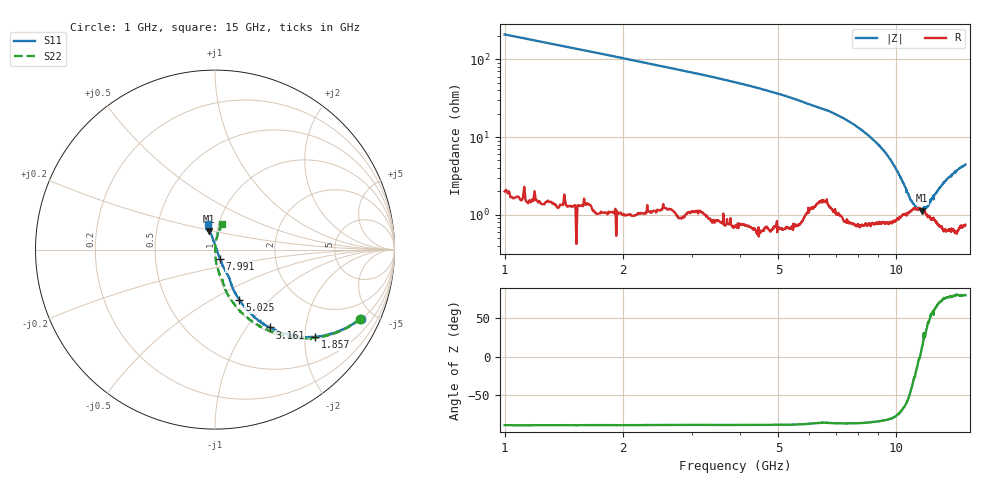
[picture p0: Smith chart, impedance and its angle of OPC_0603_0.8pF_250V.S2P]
! FILE NAME
! DATE 08/21/2012  14:12
! CORRECTED  DATA
# GHz  S  MA  R  50.00
!  FREQ  S11M  S11A  S21M  S21A  S12M  S12A  S22M  S22A
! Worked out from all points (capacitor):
!   1601 points, 1 GHz to 15 GHz, reference 50 ohm
!   read as one part in series: C = 748 fF near 1.07 GHz
!   lowest |Z| = 1.13 ohm at 11.61 GHz (marker M1)
!   series resonance near 11.49 GHz, so ESL is about 260 pH
!   S11 on the Smith chart (normalised r, x): 1 GHz: 1.06, -4.20; 1.857 GHz: 1.05, -2.26; 3.161 GHz: 1.07, -1.29; 5.025 GHz: 1.09, -0.68; 7.991 GHz: 1.05, -0.11; 15 GHz: 0.89, +0.26
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1  0.8978 -25.3  0.429 64.1  0.4288 64.0  0.8982 -25.5
1.8575  0.7409 -41.0  0.6622 48.2  0.662 48.2  0.7406 -41.6
3.16125  0.5303 -54.8  0.8365 33.2  0.8361 33.1  0.5295 -57.2
3.33625  0.5081 -56.2  0.8521 31.8  0.8514 31.8  0.5065 -58.8
5.025  0.3114 -64.1  0.9418 21.5  0.9416 21.5  0.3109 -71.2
5.6725  0.2457 -65.4  0.9599 18.6  0.9598 18.6  0.2444 -75.0
7.0375  0.1348 -64.1  0.9797 14.5  0.9792 14.4  0.132 -80.1
7.99125  0.05972 -61.9  0.9894 11.8  0.988 11.9  0.05897 -85.3
8  0.05941 -61.3  0.9893 11.8  0.988 11.8  0.05801 -86.0
8.53375  0.02257 -49.4  0.9897 10.6  0.9887 10.6  0.02034 -83.1
8.7175  0.01184 -18.4  0.9907 10.3  0.9903 10.2  0.009191 -72.6
8.83125  0.009862 9.5  0.9903 9.9  0.99 9.9  0.003107 -52.5
8.875  0.009775 23.5  0.9903 9.8  0.9899 9.8  0.001896 6.7
8.91875  0.01003 35.7  0.9899 9.7  0.9894 9.7  0.003127 57.4
9.00625  0.01222 62.6  0.9899 9.6  0.989 9.5  0.00831 76.7
9.0675  0.01479 73.1  0.9897 9.4  0.99 9.4  0.0118 80.2
9.3125  0.02736 90.4  0.9892 9.0  0.9888 9.0  0.02586 85.7
9.645  0.04435 97.4  0.9892 8.4  0.989 8.4  0.04367 83.1
10.33625  0.07381 102.6  0.9855 7.2  0.9848 7.2  0.07251 79.9
11.605  0.1073 108.3  0.9788 5.8  0.979 5.9  0.1095 76.3
12.6725  0.1242 112.2  0.9764 4.9  0.976 4.8  0.1227 77.4
15  0.1488 104.8  0.9831 3.4  0.9825 3.4  0.1494 75.2
